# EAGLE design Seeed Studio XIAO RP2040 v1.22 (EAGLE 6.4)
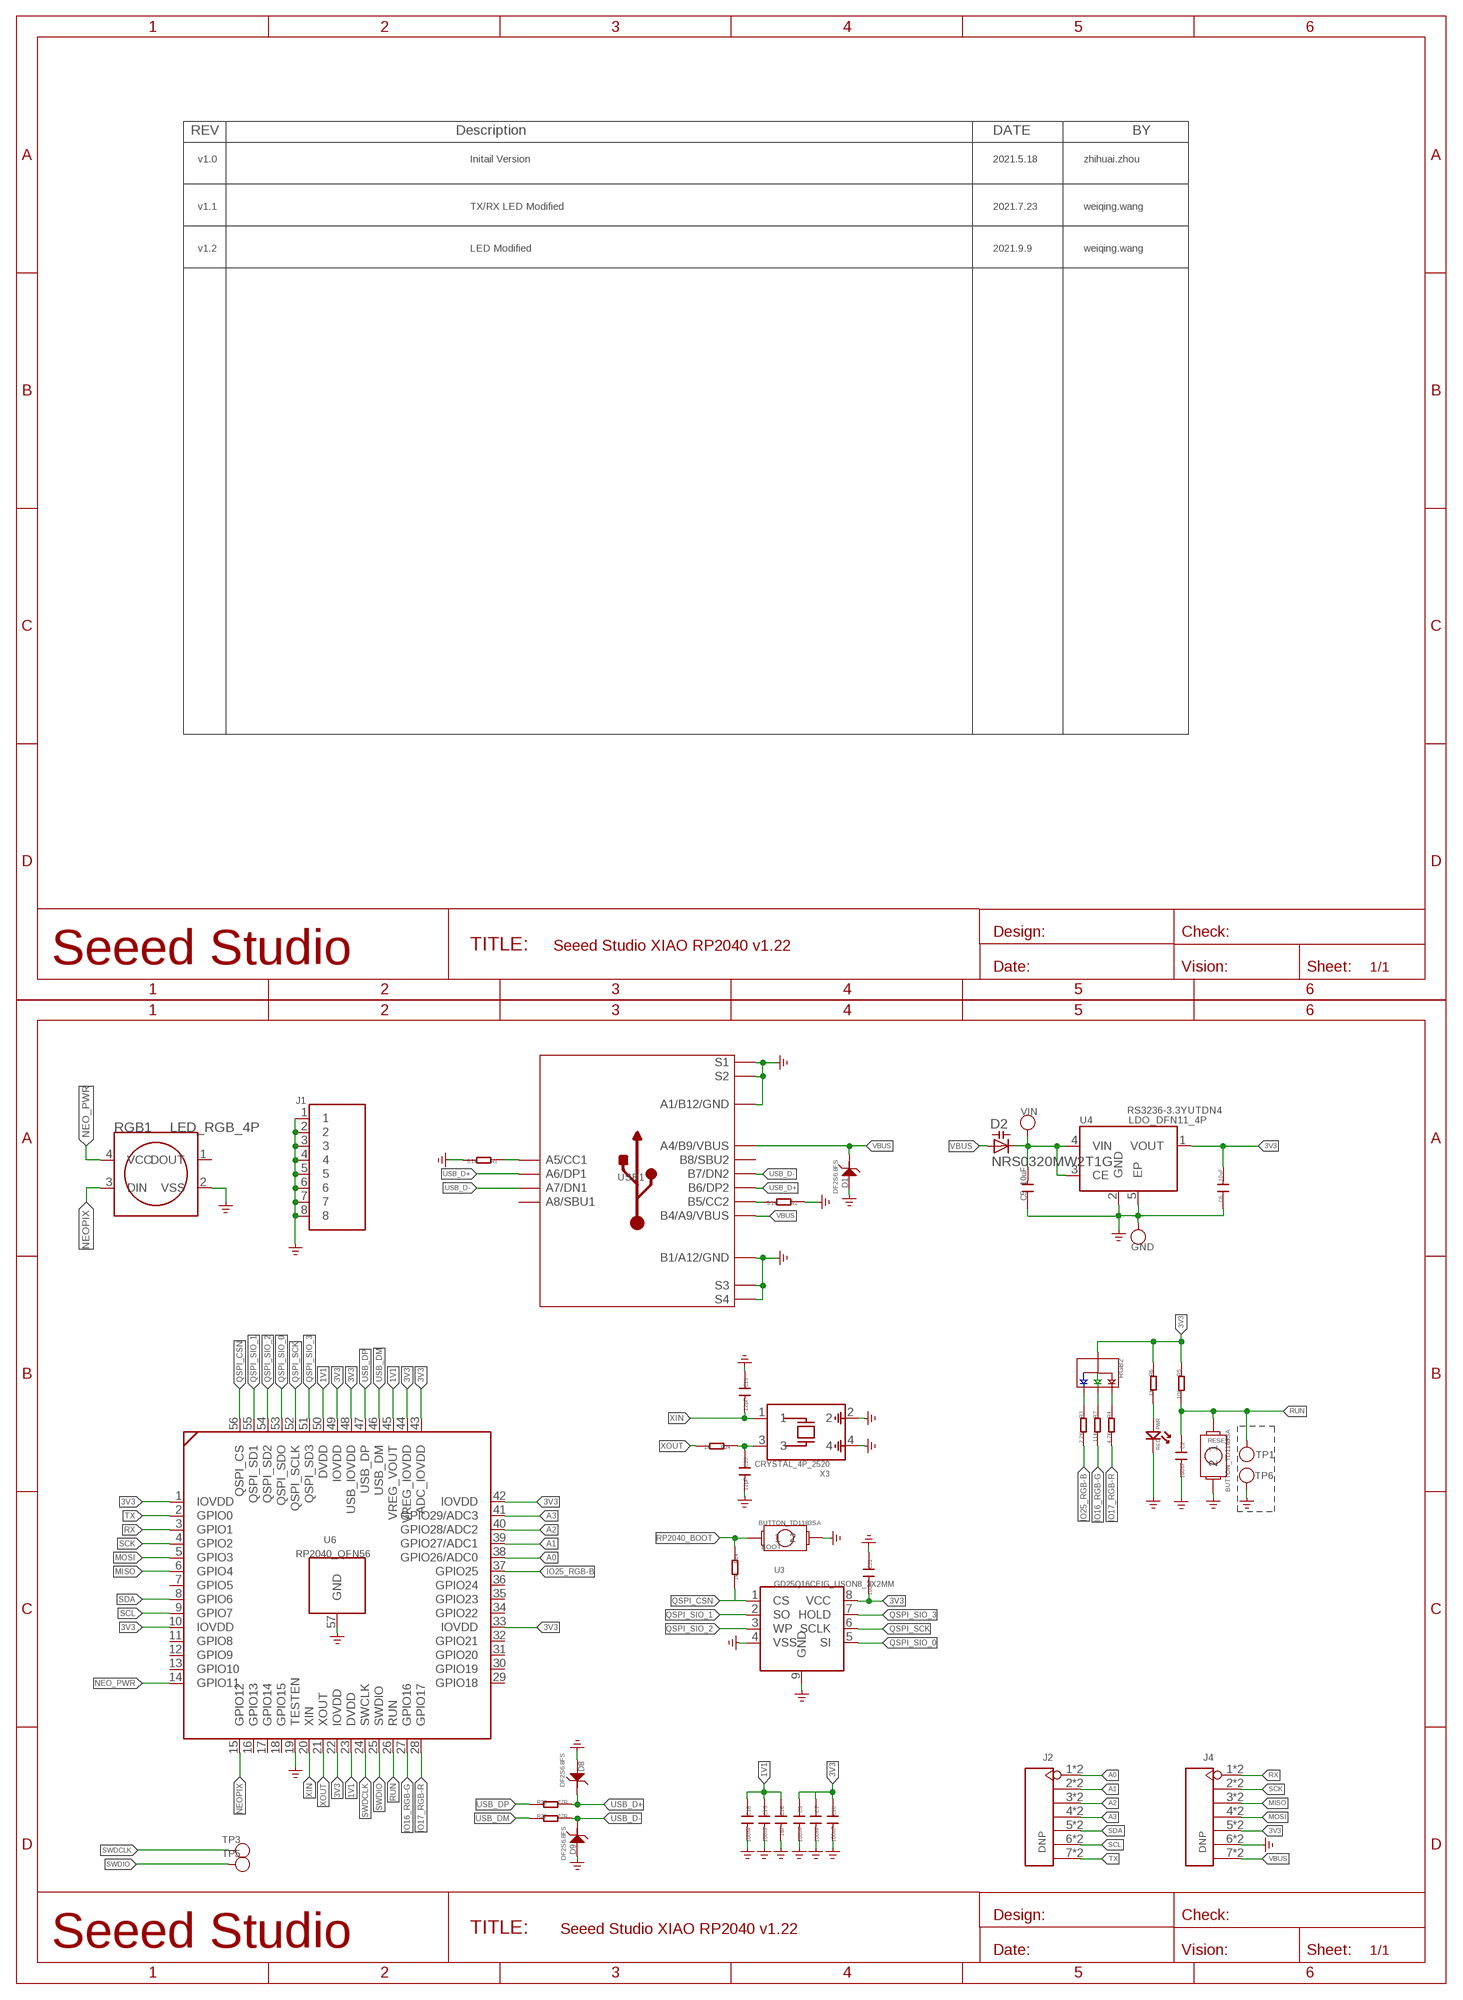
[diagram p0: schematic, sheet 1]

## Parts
BOOT  BUTTON_TD1183SA  [BUTTON_TD1183SA]
C2  100nF  CAP\0201NNS  [0201_NORMAL\NOSILK]
C3  100nF  CAP\0201NNS  [0201_NORMAL\NOSILK]
C5  10uF  C-0402  [C0402]
C6  10uF  C-0402  [C0402]
C7  100nF  CAP\0201NNS  [0201_NORMAL\NOSILK]
C10  100nF  CAP\0201NNS  [0201_NORMAL\NOSILK]
C15  100nF  CAP\0201NNS  [0201_NORMAL\NOSILK]
C16  1uF  CAP\0201NNS  [0201_NORMAL\NOSILK]
C18  100nF  CAP\0201NNS  [0201_NORMAL\NOSILK]
C19  12pF  CAP\0201NNS  [0201_NORMAL\NOSILK]
C20  12pF  CAP\0201NNS  [0201_NORMAL\NOSILK]
C21  100nF  CAP\0201NNS  [0201_NORMAL\NOSILK]
D1  DF2S6.8FS  D-ESD-2P'DF2S6.8FS'  [SOD-923]
D2  NRS0320MW2T1G  DIODE_CAPACITANCE-SOD523  [SOD523]
D8  DF2S6.8FS  D-ESD-2P'DF2S6.8FS'  [SOD-923]
D9  DF2S6.8FS  D-ESD-2P'DF2S6.8FS'  [SOD-923]
GND  TEST-POINT'4080'  [TP-80X40MIL]
J1  SHIELDING-COVER-XIAO_RP2040_PRD  [SHIELDING-COVER_XIAO_RP2040_PRD]
J2  DNP  HEADER-7P-HALF-HOLE-2.54  [H7-HALF-HOLE-2.54]
J4  DNP  HEADER-7P-HALF-HOLE-2.54  [H7-HALF-HOLE-2.54]
PWR  RED  LED-0402  [LED-0402]
R1  5.1k  R-0201  [R0201]
R2  5.1k  R-0201  [R0201]
R3  2.2K  R-0201  [R0201]
R4  4.7K  R-0201  [R0201]
R5  10k  R-0201  [R0201]
R6  1k  R-0201  [R0201]
R7  11K  R-0201  [R0201]
R14  1k  R-0201  [R0201]
R22  27R  R-0201  [R0201]
R23  27R  R-0201  [R0201]
R24  1k  R-0201  [R0201]
RESET  BUTTON_TD1183SA  [BUTTON_TD1183SA]
RGB1  LED_RGB_4P  [LED_RGB_2427]
RGB2  LED_RGB_4P-1010  [1010-4P]
TP1  TEST-POINT'4545'  [TP-D45MIL]
TP3  TEST-POINT'4545'  [TP-D45MIL]
TP5  TEST-POINT'4545'  [TP-D45MIL]
TP6  TEST-POINT'4545'  [TP-D45MIL]
U3  GD25Q16CEIG_USON8_3X2MM  [GD25Q16CEIG_USON8_3X2MM]
U4  LDO_DFN11_4P  [LDO_DFN1*1_4P]
U6  RP2040_QFN56  [RP2040_QFN56]
USB1  USB2.0-TYPE-C  [USB2.0-TYPE-C]
VIN  TEST-POINT'4080'  [TP-80X40MIL]
X3  CRYSTAL_4P_2520  [CRYSTAL_4P_2520]

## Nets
1V1: C15.1 C16.1 C18.1 U6.23(DVDD) U6.45(VREG_VOUT) U6.50(DVDD)
3V3: C3.1 C6.2 C7.1 C10.1 C21.2 J4.5 J4.17 R5.1 R6.1 RGB2.+ U3.8(VCC) U4.1(VOUT) U6.1(IOVDD) U6.10(IOVDD) U6.22(IOVDD) U6.33(IOVDD) U6.42(IOVDD) U6.43(ADC_IOVDD) U6.44(VREG_IOVDD) U6.48(USB_IOVDD) U6.49(IOVDD)
A0: J2.1 J2.13 U6.38(GPIO26/ADC0)
A1: J2.2 J2.14 U6.39(GPIO27/ADC1)
A2: J2.3 J2.15 U6.40(GPIO28/ADC2)
A3: J2.4 J2.16 U6.41(GPIO29/ADC3)
GND: BOOT.2 C2.2 C3.2 C5.1 C6.1 C7.2 C10.2 C15.2 C16.2 C18.2 C19.1 C20.2 C21.1 D1.2 D8.2 D9.2 GND.1(T) J1.1 J1.2 J1.3 J1.4 J1.5 J1.6 J1.7 J1.8 J4.6 J4.18 PWR.- R1.2 R2.1 RESET.2 RGB1.2(VSS) TP6.T U3.4(VSS) U3.9(GND) U4.2(GND) U4.5(EP) U6.19(TESTEN) U6.57(GND) USB1.A1_B12(A1/B12/GND) USB1.B1_A12(B1/A12/GND) USB1.S1 USB1.S2 USB1.S3 USB1.S4 USB1.S5(S1) USB1.S6(S2) X3.2 X3.4 ; supply symbol labelled GND_POWER
IO16_RGB-G: R7.2 U6.27(GPIO16)
IO17_RGB-R: R4.2 U6.28(GPIO17)
IO25_RGB-B: R3.2 U6.37(GPIO25)
MISO: J4.3 J4.15 U6.6(GPIO4)
MOSI: J4.4 J4.16 U6.5(GPIO3)
N$1: R1.1 USB1.A5(A5/CC1)
N$2: R2.2 USB1.B5(B5/CC2)
N$3: R3.1 RGB2.B-
N$4: R7.1 RGB2.G-
N$6: R4.1 RGB2.R-
N$8: C20.1 R24.1 X3.3
N$16: PWR.+ R6.2
NEO_PWR: RGB1.4(VCC) U6.14(GPIO11)
NEOPIX: RGB1.3(DIN) U6.15(GPIO12)
QSPI_CSN: R14.2 U3.1(CS) U6.56(QSPI_CS)
QSPI_SCK: U3.6(SCLK) U6.52(QSPI_SCLK)
QSPI_SIO_0: U3.5(SI) U6.53(QSPI_SDO)
QSPI_SIO_1: U3.2(SO) U6.55(QSPI_SD1)
QSPI_SIO_2: U3.3(WP) U6.54(QSPI_SD2)
QSPI_SIO_3: U3.7(HOLD) U6.51(QSPI_SD3)
RP2040_BOOT: BOOT.1 R14.1
RUN: C2.1 R5.2 RESET.1 TP1.T U6.26(RUN)
RX: J4.1 J4.13 U6.3(GPIO1)
SCK: J4.2 J4.14 U6.4(GPIO2)
SCL: J2.6 J2.18 U6.9(GPIO7)
SDA: J2.5 J2.17 U6.8(GPIO6)
SWDCLK: TP3.T U6.24(SWCLK)
SWDIO: TP5.T U6.25(SWDIO)
TX: J2.7 J2.19 U6.2(GPIO0)
USB_D+: D8.1 R23.2 USB1.A6(A6/DP1) USB1.B6(B6/DP2)
USB_D-: D9.1 R22.2 USB1.A7(A7/DN1) USB1.B7(B7/DN2)
USB_DM: R22.1 U6.46(USB_DM)
USB_DP: R23.1 U6.47(USB_DP)
VBUS: D1.1 D2.A J4.7 J4.19 USB1.A4_B9(A4/B9/VBUS) USB1.B4_A9(B4/A9/VBUS)
VIN: C5.2 D2.C U4.3(CE) U4.4(VIN) VIN.1(T)
XIN: C19.2 U6.20(XIN) X3.1
XOUT: R24.2 U6.21(XOUT)
Unconnected: RGB1.1(DOUT) U6.7(GPIO5) U6.11(GPIO8) U6.12(GPIO9) U6.13(GPIO10) U6.16(GPIO13) U6.17(GPIO14) U6.18(GPIO15) U6.29(GPIO18) U6.30(GPIO19) U6.31(GPIO20) U6.32(GPIO21) U6.34(GPIO22) U6.35(GPIO23) U6.36(GPIO24) USB1.A8(A8/SBU1) USB1.B8(B8/SBU2)

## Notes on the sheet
- v1.0 | Initail Version | 2021.5.18 | zhihuai.zhou
- v1.1 | TX/RX LED Modified | 2021.7.23 | weiqing.wang
- v1.2 | LED Modified | 2021.9.9 | weiqing.wang
- RS3236-3.3YUTDN4

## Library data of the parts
BOOT RESET = BUTTON_TD1183SA:BUTTON_TD1183SA: 德艺隆:TD-1183SA/311020740
C2 C3 C7 C10 C15 C16 C18-C21 = Seeed-Discrete:CAP: Ceramic Capacitors
C5 C6 = XIAO RP2040 PRD v1.0:C*: Ceramic Capacitors
D1 D8 D9 = Discrete-new:D-ESD-2P: SOD-923:304060009;SOD-123:304060001
D2 = XIAO RP2040 PRD v1.0:DIODE_CAPACITANCE-: Capacity DIODE
GND VIN = Discrete-new:TEST-POINT
J1 = XIAO RP2040 PRD v1.0:SHIELDING-COVER-XIAO_RP2040_PRD
J2 J4 = Connector-new:HEADER-7P-HALF-HOLE
PWR = Discrete-small:LED
R1-R7 R14 R22-R24 = XIAO RP2040 PRD v1.0:R*
RGB1 = XIAO RP2040 PRD v1.0:LED_RGB_4P
RGB2 = Seeed-Discrete:LED_RGB_4P
TP1 TP3 TP5 TP6 = Discrete-new:TEST-POINT; PARTNO: DNP
U3 = FLASH_GD25Q16CEIG_2:GD25Q16CEIG_USON8_3X2MM
U4 = LDO_DFN1X1_4P:LDO_DFN1*1_4P
U6 = RP2040_QFN56:RP2040_QFN56
USB1 = USB C:USB2.0-TYPE-C
X3 = CRYSTAL_4P:CRYSTAL_4P_2520

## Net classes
1 power: width 0.152 mm, drill 0.152 mm, clearance 0.152 mm
2 gnd: width 0.152 mm, drill 0.152 mm, clearance 0.152 mm
3 usbvcc: width 0.152 mm, drill 0.152 mm, clearance 0.152 mm

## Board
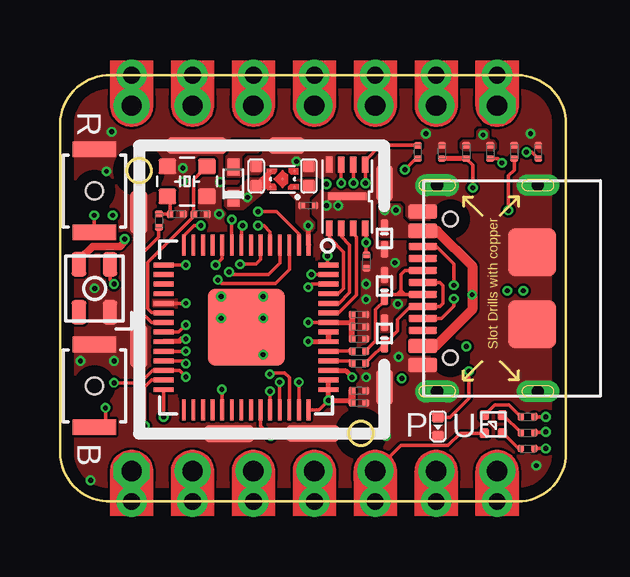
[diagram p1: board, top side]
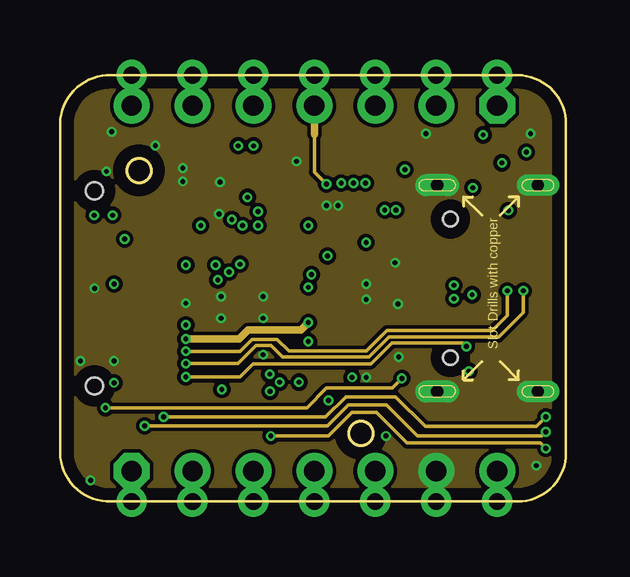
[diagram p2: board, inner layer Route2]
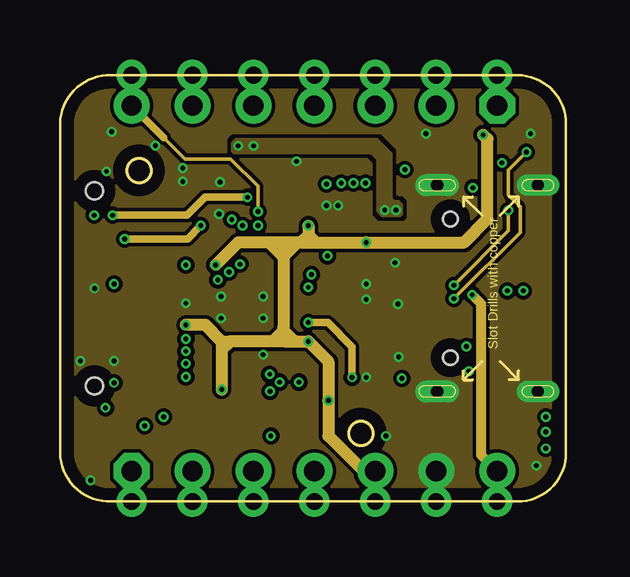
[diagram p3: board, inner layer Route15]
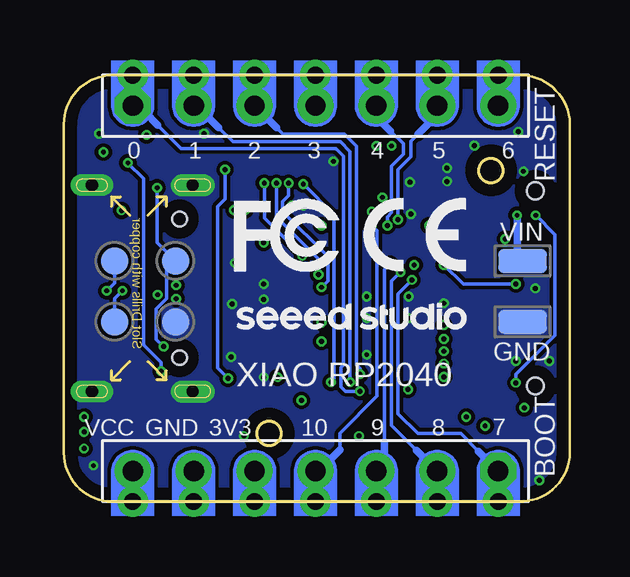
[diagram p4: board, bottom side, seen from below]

Size 21.1 x 17.78 mm. Coordinates in mm from the lower left corner, seen from the top.
Outline: 2.13,0 19.07,0 arc90 21.1,2.03 21.1,15.75 arc90 19.07,17.78 2.13,17.78 arc90 0,15.75 0,2.03 arc90 2.13,0
Copper layers (1+2*15+16): Top 0.035mm / dielectric 0.2mm / Route2 0.0175mm / dielectric 1.1mm / Route15 0.0175mm / dielectric 0.2mm / Bottom 0.035mm
Design rules "SeeedStudio_2layer_DRU_no_angle_20140221 *": minimum track width 1mil, minimum drill 8mil, track to track 4mil, track to pad 4mil, pad to pad 6mil, via to via 4mil, smd to smd 0mil, copper to edge 20mil, drill to drill 10mil, minimum pad ring 4mil, minimum via ring 4mil, stop-mask expansion 2mil, vias tented up to drill 25mil, thermal gap 0mil
tRestrict: area 4.9,4.3 to 10.6,10.2

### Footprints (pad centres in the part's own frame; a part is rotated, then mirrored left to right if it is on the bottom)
BUTTON_TD1183SA = smd 0.65 x 1.8: 1 -1.725,0; 2 1.725,0 | hole 0.7: 0,0
0201_NORMAL\NOSILK = smd 0.279 x 0.318: 1 -0.279,0; 2 0.279,0
C0402 = smd 0.508 x 0.508: 1 -0.406,0; 2 0.406,0
SOD-923 = smd 0.7 x 0.3: 1 -0.45,0; 2 0.45,0
SOD523 = smd 0.7 x 0.5: A 0.7,0; C -0.6,0
TP-80X40MIL = smd 2.032 x 1.016: 1 0,0
SHIELDING-COVER_XIAO_RP2040_PRD = smd 0.7 x 1.778: 1 -4.953,3.556; 2 -4.953,-2.032 | smd 2.032 x 0.7: 3 -1.18,-5.673 | smd 2.2 x 0.7: 4 2.29,-5.668 | smd 0.7 x 1.5: 5 5.283,-3.737; 6 5.283,4.772 | smd 1.5 x 0.7: 7 1.216,6.332 | smd 2.5 x 0.7: 8 -2.54,6.332 | hole 1: -4.953,5.3; 4.3,-5.672
H7-HALF-HOLE-2.54 = drill 0.85 pad 1.5 octagon: 1 0,7.62 | drill 0.85 pad 1.5: 2 0,5.08; 3 0,2.54; 4 0,0; 5 0,-2.54; 6 0,-5.08; 7 0,-7.62 | drill 0.7 pad 1.27: 13 -1.27,7.62; 14 -1.27,5.08; 15 -1.27,2.54; 16 -1.27,0; 17 -1.27,-2.54; 18 -1.27,-5.08; 19 -1.27,-7.62
LED-0402 = smd 0.385 x 0.508: + -0.383,0; - 0.383,0
R0201 = smd 0.279 x 0.318: 1 -0.279,0; 2 0.279,0
LED_RGB_2427 = smd 1 x 0.6: 1 1,-0.65; 2 1,0.65; 3 -1,0.65; 4 -1,-0.65
1010-4P = smd 0.4 x 0.4: + 0.375,0.375; B- -0.375,0.375; G- -0.375,-0.375; R- 0.375,-0.375
TP-D45MIL = smd 1.143 x 1.143: T 0,0
GD25Q16CEIG_USON8_3X2MM = smd 0.65 x 0.3: 1 -1.33,0.75; 2 -1.33,0.25; 3 -1.33,-0.25; 4 -1.33,-0.75; 5 1.33,-0.75; 6 1.33,-0.25; 7 1.33,0.25; 8 1.33,0.75 | smd 0.3 x 1.6: 9 0,0
LDO_DFN1*1_4P = smd 0.1 x 0.1: 1 -0.33,-0.5; 2 0.33,-0.5; 3 0.33,0.51; 4 -0.33,0.5; 5 0,0
RP2040_QFN56 = smd 0.875 x 0.2: 1 -3.438,2.6; 2 -3.438,2.2; 3 -3.438,1.8; 4 -3.438,1.4; 5 -3.438,1; 6 -3.438,0.6; 7 -3.438,0.2; 8 -3.438,-0.2; 9 -3.438,-0.6; 10 -3.438,-1; 11 -3.438,-1.4; 12 -3.438,-1.8; 13 -3.438,-2.2; 14 -3.438,-2.6; 29 3.438,-2.6; 30 3.438,-2.2; 31 3.438,-1.8; 32 3.438,-1.4; 33 3.438,-1; 34 3.438,-0.6; 35 3.438,-0.2; 36 3.438,0.2; 37 3.438,0.6; 38 3.438,1; 39 3.438,1.4; 40 3.438,1.8; 41 3.438,2.2; 42 3.438,2.6 | smd 0.2 x 0.875: 15 -2.6,-3.438; 16 -2.2,-3.438; 17 -1.8,-3.438; 18 -1.4,-3.438; 19 -1,-3.438; 20 -0.6,-3.438; 21 -0.2,-3.438; 22 0.2,-3.438; 23 0.6,-3.438; 24 1,-3.438; 25 1.4,-3.438; 26 1.8,-3.438; 27 2.2,-3.438; 28 2.6,-3.438; 43 2.6,3.438; 44 2.2,3.438; 45 1.8,3.438; 46 1.4,3.438; 47 1,3.438; 48 0.6,3.438; 49 0.2,3.438; 50 -0.2,3.438; 51 -0.6,3.438; 52 -1,3.438; 53 -1.4,3.438; 54 -1.8,3.438; 55 -2.2,3.438; 56 -2.6,3.438 | smd 3.2 x 3.2: 57 0,0
USB2.0-TYPE-C = smd 1.2 x 0.6: A1_B12 0.05,3.2; A4_B9 0.05,2.4; B1_A12 0.05,-3.2; B4_A9 0.05,-2.4 | smd 1.2 x 0.3: A5 0.05,1.25; A6 0.05,0.25; A7 0.05,-0.25; A8 0.05,-1.25; B5 0.05,-1.75; B6 0.05,-0.75; B7 0.05,0.75; B8 0.05,1.75 | drill 0.508 pad 0.889 long: S1 -4.75,4.3; S2 -4.75,-4.3 | drill 0.508 pad 0.914 long: S3 -0.55,4.3; S4 -0.55,-4.3 | smd 2 x 2: S5 -4.5,1.5; S6 -4.5,-1.5 | hole 0.6: -1.1,-2.89; -1.1,2.89
CRYSTAL_4P_2520 = smd 0.75 x 0.65: 1 -0.825,-0.625; 2 0.825,-0.625; 3 0.825,0.625; 4 -0.825,0.625

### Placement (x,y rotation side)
BOOT  1.44,4.83 90 top
C2  15.93,14.58 90 top
C3  10.36,12.34 0 top
C5  8.18,13.58 270 top
C6  10.38,13.58 270 top
C7  12.46,4.62 0 top
C10  12.46,4.11 0 top
C15  12.46,7.8 0 top
C16  12.46,6.78 0 top
C18  12.46,7.29 0 top
C19  5.87,11.97 180 top
C20  4.87,11.97 0 top
C21  12.78,10.01 90 top
D1  13.53,10.97 270 top
D2  7.23,13.25 90 top
D8  13.53,8.99 90 top
D9  13.53,7.01 90 top
GND  1.97,7.49 0 bottom
J1  8.25,8.51 0 top
J2  10.61,16.51 270 top
J4  10.61,1.27 90 top
PWR  15.77,3.12 270 top
R1  19.94,14.58 90 top
R2  18.94,14.58 270 top
R3  19.5,2.21 0 top
R4  19.5,3.53 0 top
R5  16.93,14.58 270 top
R6  17.94,14.58 270 top
R7  19.5,2.87 0 top
R14  14.93,14.58 90 top
R22  12.46,5.77 0 top
R23  12.46,6.27 0 top
R24  4.12,11.71 270 top
RESET  1.44,12.95 90 top
RGB1  1.44,8.89 270 top
RGB2  18.08,3.22 180 top
TP1  16.45,10.03 0 bottom
TP3  18.99,7.49 0 bottom
TP5  18.99,10.03 0 bottom
TP6  16.45,7.49 0 bottom
U3  11.98,12.73 270 top
U4  9.29,13.44 90 top
U6  7.76,7.26 270 top
U$4  [LOGO-SEEED-NEW-1X9.6MM]  13.91,7.11 0 bottom
USB1  15.18,8.89 180 top
VIN  1.97,10.03 180 bottom
X3  5.3,13.35 180 top

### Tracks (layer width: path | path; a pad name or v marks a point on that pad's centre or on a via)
1V1  (via drill 0.2 pad 0.41)
  Top 0.152: v10.36,7.46 U6.50
  Top 0.203: U6.50 12.18,7.46 C18.1 | U6.23 4.34,6.68 4.97,6.68 5.07,6.78 v5.25,6.78 | U6.45 11.9,5.46 v12.18,5.18
  Top 0.254: C15.1 C18.1 C16.1
  Route2 0.305: v5.25,6.78 7.48,6.78 7.85,7.16 10.05,7.16 v10.36,7.46
  Route15 0.305: v12.18,5.18 12.18,6.45 11.17,7.46 v10.36,7.46
3V3  (via drill 0.2 pad 0.41)
  Top 0.152: U6.22 4.95,7.06 v5.25,7.37 | v11.19,4.22 10.8,3.83 U6.42 | U3.8 12.77,11.36 v12.77,10.8 12.77,10.3 C21.2 | v6.75,4.67 6.76,4.66 U6.33 | v6.49,9.87 6.76,10.14 U6.10 | RGB2.+ 16.69,2.85 16.18,2.34 14.22,2.34 J4.5
  Top 0.203: U6.48 U6.49 11.2,6.68 v10.36,6.68 | U6.44 U6.43 v11.19,4.22 12.08,4.22 C10.1 | U6.42 10.38,3.84 | U6.1 v10.36,11.51
  Top 0.254: J4.5 J4.17
  Top 0.305: C10.1 C7.1
  Route15 0.305: 8.59,10.8 9.26,10.14 9.31,10.14 9.37,10.14 10.04,10.8 | 8.59,6.68 8.73,6.68 9.31,7.26 9.85,6.73 9.85,6.68
  Route15 0.508: 9.34,6.68 9.85,6.68 v10.36,6.68 11.19,5.84 v11.19,4.22 11.19,2.73 12.66,1.27 J4.5 | 9.34,6.68 8.59,6.68 7.1,6.68 | 6.75,6.68 7.1,6.68 | 10.36,10.8 10.67,10.8 | v10.36,11.51 10.36,11.12 | 10.36,11.12 10.36,10.8 | 10.04,10.8 10.36,10.8 | 10.04,10.8 9.31,10.8 | 9.31,10.8 8.59,10.8 7.43,10.8 v6.49,9.87 | 7.1,6.68 6.75,6.33 | 10.04,10.8 10.36,11.12 | 10.36,11.12 10.67,10.8 | 9.31,10.8 9.31,10.14 9.31,7.26 9.31,6.71 9.34,6.68 | 6.75,6.68 6.75,6.33 | v17.65,15.29 17.82,15.11 17.82,11.77 16.85,10.8 v12.77,10.8 10.67,10.8 | v5.25,7.37 6.06,7.37 6.75,6.68 | 6.75,6.33 v6.75,4.67
  pour Top: 9.5,13.06 9.9,13.45 10.63,13.45 10.72,13.36 10.72,12.99 10.38,12.65 10.38,11.89 10.62,11.65 10.62,11.38 10.51,11.26 10.22,11.26 9.85,11.63 9.85,12.55 9.5,12.89
  pour Top: 17.3,15.07 16.79,15.07 16.67,14.95 16.67,14.76 16.79,14.63 18.09,14.63 18.22,14.76 18.22,14.94 18.09,15.06 17.99,15.06 17.91,15.14 17.91,15.43 17.81,15.53 17.47,15.53 17.37,15.43 17.37,15.14
A0  (via drill 0.2 pad 0.41)
  Top 0.152: v8.76,4.6 U6.38
  Top 0.254: J2.1 J2.13
  Bottom 0.152: 17.19,15.7 16.21,14.72 9.75,14.72 9.44,14.41 9.44,5.7 9.54,5.6 9.54,4.79 9.35,4.6 9,4.6 v8.76,4.6
  Bottom 0.305: 17.19,15.7 17.72,16.23 17.95,16.23 J2.1
A1  (via drill 0.2 pad 0.41)
  Top 0.152: v9.16,4.98 U6.39
  Top 0.254: J2.2 J2.14
  Bottom 0.102: J2.2 15.69,16
  Bottom 0.152: 14.65,15.6 14.05,15 9.57,15 9.16,14.59 v9.16,4.98
  Bottom 0.305: 14.65,15.6 15.08,16.03 15.66,16.03 15.69,16
A2  (via drill 0.2 pad 0.41)
  Top 0.152: U6.40 9.57,5.17 9.36,5.37 8.81,5.37 v8.75,5.31
  Top 0.254: J2.3 J2.15
  Bottom 0.152: 12.34,15.7 12.34,15.65 | v8.75,5.31 8.75,5.55 8.9,5.7 8.9,14.82 9.39,15.32 11.96,15.32 12.24,15.6
  Bottom 0.305: J2.3 12.34,15.7 12.24,15.6
A3  (via drill 0.2 pad 0.41)
  Top 0.152: v9.96,4.98 U6.41
  Top 0.254: J2.4 J2.16
  Route2 0.152: 10.61,15.32 10.61,13.74 v11.12,13.23
  Route2 0.305: J2.4 10.61,15.32
  Bottom 0.152: v9.96,4.98 9.83,5.11 9.83,11.95 v11.12,13.23
GND  (via drill 0.2 pad 0.41)
  Top 0.152: v5.25,8.27 v5.25,8.26 U6.19
  Top 0.305: U6.57 7.76,6.83 v8.48,6.12
  other vias: 8.48,7.65 6.72,7.65 8.48,8.55 1.44,8.89 0.86,5.87 2.25,5.87 1.94,13.77 2.15,15.42 3.98,14.85 6.68,13.32 11.12,12.34 11.6,12.34 12.77,8.43 12.77,9.07 12.77,5.18 1.28,0.89 19.87,1.5 13.59,2.73 19.63,15.34 15.26,15.34 6.72,8.55 5.12,13.91 9.86,14.19 14.13,6.03 14.09,8.24 13.98,9.96 6.63,11.99 5.12,13.35
  pour Top (rank 3, no thermals): -0.19,17.93 21.51,17.93 21.53,17.91 21.53,-0.28 3.88,-0.28 3.88,-0.91 2.08,-0.91 2.08,-0.25 -0.21,-0.25
  pour Route2 (isolate 0.152, rank 6, no thermals): -0.19,17.93 21.51,17.93 21.53,17.91 21.53,-0.28 3.88,-0.28 3.85,-1.24 2.08,-1.24 2.08,-0.25 -0.21,-0.25
  pour Route15 (isolate 0.152, rank 6, no thermals): -0.19,17.93 21.51,17.93 21.53,17.91 21.53,-0.28 3.88,-0.28 3.85,-1.57 2.08,-1.57 2.08,-0.25 -0.21,-0.25
  pour Bottom (isolate 0.152, rank 6, no thermals): -0.19,17.93 21.51,17.93 21.53,17.91 21.53,-0.28 3.88,-0.28 3.85,-1.93 2.08,-1.93 2.08,-0.25 -0.21,-0.25
IO16_RGB-G  (via drill 0.2 pad 0.41)
  Top 0.152: U6.27 3.82,5.06 3.54,4.78 v3.54,3.15 | R7.2 20.23,2.87 v20.26,2.91
  Route2 0.152: v3.54,3.15 11.16,3.15 12.03,4.02 13.62,4.02 14.9,2.74 20.1,2.74 v20.26,2.91
IO17_RGB-R  (via drill 0.2 pad 0.41)
  Top 0.152: U6.28 v4.33,3.54 v4.32,3.53 | R4.2 v20.26,3.54 v20.26,3.53
  Route2 0.152: v4.32,3.53 11.08,3.53 11.92,4.37 13.99,4.37 15.23,3.12 19.86,3.12 v20.26,3.53
IO25_RGB-B  (via drill 0.2 pad 0.41)
  Top 0.152: U6.37 8.36,3.16 v8.79,2.73 | R3.2 v20.26,2.21
  Route2 0.152: v8.79,2.73 11.19,2.73 12.17,3.71 13.2,3.71 14.47,2.44 20.03,2.44 v20.26,2.21
MISO  (via drill 0.2 pad 0.41)
  Top 0.152: U6.6 8.37,10.69 8.37,10.08 8.19,9.9 v7.51,9.9
  Top 0.254: J4.3 J4.15
  Bottom 0.152: v7.51,9.9 7.74,9.67 7.74,2.49
  Bottom 0.305: J4.3 7.74,1.6 7.74,2.49
MOSI  (via drill 0.2 pad 0.41)
  Top 0.152: U6.5 8.76,11.24 8.5,11.51 v8.26,11.51
  Top 0.254: J4.4 J4.16
  Bottom 0.152: 9.59,2.15 9.59,2.85 8.04,4.39 8.04,11.29 v8.26,11.51
  Bottom 0.305: 9.59,2.15 10.47,1.27 J4.4
N$1  (via drill 0.2 pad 0.41)
  Top 0.152: USB1.A5 15.91,7.64 16.43,8.15 v16.43,8.46 | R1.1 19.68,14.57 v19.45,14.57
  Route15 0.152: v16.43,8.46 19.19,11.23 19.19,12.29 18.7,12.79 18.7,13.82 v19.45,14.57
N$2  (via drill 0.2 pad 0.41)
  Top 0.152: USB1.B5 15.69,10.64 16.43,9.91 v16.43,9.02 | v18.7,12.14 18.7,13.59 18.94,13.83 R2.2
  Route15 0.152: v16.43,9.02 18.7,11.29 v18.7,12.14
N$3
  Top 0.152: RGB2.B- 18.48,2.85 19.12,2.21 R3.1
N$4
  Top 0.152: RGB2.G- 18.5,3.6 R7.1
N$6
  Top 0.152: 17.7,3.64 RGB2.R- 18.14,4.04 18.72,4.04 R4.1
N$8
  Top 0.152: R24.1 4.57,11.99 C20.1 4.59,12.61 X3.3
N$16  (via drill 0.2 pad 0.41)
  Top 0.152: v18.43,14.12 18.25,14.3 R6.2 | v17.05,5.44 17.05,4.31 16.25,3.51 PWR.+
  Bottom 0.152: v18.43,14.12 17.77,13.46 17.77,6.53 17.05,5.8 v17.05,5.44
NEO_PWR  (via drill 0.2 pad 0.41)
  Top 0.152: RGB1.4 0.79,10.07 | U6.14 5.16,11.08 5.59,11.51 v5.87,11.51
  Top 0.305: 0.79,10.07 1.37,10.64 2.5,10.64 2.7,10.84 v2.7,10.95
  Route15 0.305: v2.7,10.95 5.31,10.95 v5.87,11.51
NEOPIX  (via drill 0.2 pad 0.41)
  Top 0.152: v5.25,9.87 U6.15 | 2.09,9.49 RGB1.3 2.09,9.23 v2.25,9.07
  Bottom 0.152: v2.25,9.07 4.45,9.07 v5.25,9.87
QSPI_CSN  (via drill 0.2 pad 0.41)
  Top 0.152: v11.16,10.25 11.15,10.24 11.15,9.92 U6.56 | R14.2 13.37,14.86 12.73,14.22 U3.1 12.74,14.04 v12.74,13.28
  Bottom 0.152: v11.16,10.25 12.74,11.83 v12.74,13.28
QSPI_SCK
  Top 0.152: U3.6 11.73,11.05 12.08,10.7 12.08,8.72 11.63,8.26 U6.52
QSPI_SIO_0
  Top 0.152: 11.28,11.23 11.28,11.35 U3.5 11.23,11.01 11.83,10.41 11.83,8.89 11.6,8.66 U6.53
QSPI_SIO_1  (via drill 0.2 pad 0.41)
  Top 0.152: v10.48,9.47 v10.49,9.46 U6.55 | v12.24,13.28 U3.2
  Bottom 0.152: 12.24,13.31 v12.24,13.28 12.24,11.86 10.48,10.11 v10.48,9.47
QSPI_SIO_2  (via drill 0.2 pad 0.41)
  Top 0.152: v11.73,13.28 U3.3 | v10.36,8.94 10.48,9.06 U6.54
  Bottom 0.152: v11.73,13.28 11.73,12.76 11.98,12.5 11.98,12.09 10.1,10.21 10.1,9.2 v10.36,8.94
QSPI_SIO_3
  Top 0.152: U6.51 11.61,7.86 12.37,8.62 12.37,11.04 12.23,11.18 U3.7
RP2040_BOOT  (via drill 0.2 pad 0.41)
  Top 0.152: R14.1 14.84,14.3 v14.38,13.84 | v1.9,3.91 1.9,2.97 1.95,2.92 1.62,2.92 BOOT.1
  Route2 0.152: v1.9,3.91 10.29,3.91 11.12,4.74 13.86,4.74 v14.25,5.13
  Bottom 0.152: v14.25,5.13 14.7,5.58 14.7,12.29 14.38,12.61 v14.38,13.84
RUN  (via drill 0.2 pad 0.41)
  Top 0.152: RESET.1 1.43,11.24 v1.43,11.94 | R5.2 17.21,14.02 v17.21,13.08 | v2.25,4.95 3.35,4.95 3.86,5.46 U6.26 4.98,5.46 v5.25,5.19
  Top 0.203: R5.2 C2.1
  Route2 0.152: v16.95,6.46 16.81,6.6 13.84,6.6 12.97,5.74 8.06,5.74 7.51,5.19 v5.25,5.19
  Bottom 0.152: v17.21,13.08 17.21,10.79 TP1.T 16.81,9.68 16.81,8.46 17.25,8.02 17.25,6.77 v16.95,6.46 | v1.43,11.94 0.63,11.14 0.63,6.93 2.25,5.31 v2.25,4.95
RX  (via drill 0.2 pad 0.41)
  Top 0.152: v6.58,9.25 6.74,9.09 8.98,9.09 9.57,9.68 U6.3 | J4.1 2.99,0.33
  Top 0.254: J4.1 J4.13
  Bottom 0.152: 3.81,2.09 4.55,2.83 6.34,2.83 7.17,3.66 7.17,8.66 v6.58,9.25 | v6.58,9.25
  Bottom 0.305: J4.1 3.81,2.09
SCK  (via drill 0.2 pad 0.41)
  Top 0.152: v7.06,9.57 7.16,9.47 8.7,9.47 9.17,9.94 9.17,10.69 U6.4
  Top 0.254: J4.2 J4.14
  Bottom 0.152: 6.4,2.14 7.43,3.18 7.43,9.2 v7.06,9.57
  Bottom 0.305: J4.2 6.4,2.14
SCL  (via drill 0.2 pad 0.41)
  Top 0.152: U6.9 v7.16,11.76 v7.17,11.76
  Top 0.254: J2.6 J2.18
  Bottom 0.152: v7.17,11.76 7.17,13.84 6.63,14.38 6.63,15.02 6.33,15.33
  Bottom 0.305: J2.6 5.53,16.13 6.33,15.33
SDA  (via drill 0.2 pad 0.41)
  Top 0.152: U6.8 7.56,11.46 v7.61,11.51
  Top 0.254: J2.5 J2.17
  Bottom 0.152: v7.61,11.51 7.61,11.87 7.43,12.05 7.43,14 6.95,14.48 6.95,14.92 7.49,15.46
  Bottom 0.305: J2.5 8.07,16.04 7.49,15.46
SWDCLK  (via drill 0.2 pad 0.41)
  Top 0.152: v5.25,6.27 U6.24
  Route2 0.152: v5.25,6.27 7.52,6.27 8.01,6.76 9.05,6.76 9.54,6.27 10.14,6.27 12.78,6.27 13.63,7.13 18.03,7.13 18.66,7.76 v18.66,8.79
  Bottom 0.152: v18.66,8.79 18.99,8.46 TP3.T
SWDIO  (via drill 0.2 pad 0.41)
  Top 0.152: v5.25,5.75 5.14,5.86 U6.25
  Route2 0.152: v5.25,5.75 7.43,5.75 8.17,6.5 8.79,6.5 9.28,6.02 12.88,6.02 13.72,6.86 18.29,6.86 19.32,7.89 v19.32,8.79
  Bottom 0.152: v19.32,8.79 18.99,9.12 TP5.T
TX  (via drill 0.2 pad 0.41)
  Top 0.152: U6.2 9.96,11.15 9.02,12.09 v8.26,12.09 | 2.99,17.34 J2.19
  Top 0.381: J2.7 2.99,17.34
  Route15 0.152: v8.26,12.09 8.26,13.14 7.12,14.29 5.21,14.29 4.32,15.18
  Route15 0.305: J2.7 4.32,15.18
USB_D+
  Top 0.102: USB1.A6
  Top 0.152: USB1.B6 14.38,9.64 14.22,9.47 14.22,8.8 | R23.2 12.91,6.45 12.92,6.45 13.16,6.69 13.16,8 13.53,8.37 D8.1 13.62,8.54 13.72,8.64 | 13.63,8.64 13.72,8.64 | 13.72,8.64 13.92,8.64 14.05,8.64 | 14.05,8.64 14.22,8.64 | 14.22,8.64 14.38,8.64 | 14.38,8.64 USB1.A6 | 14.22,8.8 14.22,8.64 | 14.05,8.64 14.22,8.8 | 14.22,8.8 14.38,8.64
USB_D-
  Top 0.152: USB1.A7 15.84,9.14 15.97,9.02 15.97,8.26 15.85,8.14 USB1.B7 15.12,8.13 14.62,8.13 14.08,7.59 14.08,7.11 D9.1 12.92,5.94 12.91,5.94 R22.2
USB_DM
  Top 0.152: U6.46 12.09,5.86 R22.1
USB_DP
  Top 0.152: R23.1 11.2,6.27 U6.47
VBUS  (via drill 0.2 pad 0.41)
  Top 0.254: J4.7 J4.19
  Top 0.406: USB1.B4_A9 15.73,11.29 17.19,9.83 v17.19,8.62 17.19,8 15.69,6.5 15.14,6.5 USB1.A4_B9
  Route15 0.406: v17.19,8.62 17.56,8.26 17.56,1.94 J4.7
  other vias: 13.54,12.15 14.01,12.15 7.43,14.83 8.07,14.83
  pour Bottom (isolate 0.254, no thermals): 18.38,1.37 18,0.99 17.72,0.99
  pour Top: 13.38,11.01 15.64,11.01 15.69,11.06 15.69,11.53 15.65,11.57 14.53,11.57 14.31,11.8 14.31,12.08 14.31,12.28 14.18,12.41 13.42,12.41 13.28,12.27 13.28,11.98 13.28,11.11
  pour Top: 6.96,13.54 7.54,13.54 7.59,13.59 7.59,14.4 7.74,14.55 8.26,14.55 8.35,14.64 8.35,14.97 8.25,15.07 7.23,15.07 6.9,14.74 6.9,13.6
  pour Route15: 7.27,15.09 7.13,14.95 7.13,14.62 7.24,14.5 7.5,14.5 12.97,14.5 13.19,14.29 13.19,12.1 13.4,11.89 14.2,11.89 14.31,11.99 14.31,12.38 14.14,12.55 13.96,12.55 13.87,12.64 13.87,14.5 13.4,14.97 13.24,15.14 7.4,15.14 7.32,15.14
VIN  (via drill 0.2 pad 0.41)
  Top 0.152: C5.2 8.21,13.2 | C5.2 8.43,13.41 8.49,13.41 | 8.62,13.29 8.49,13.41 | 8.62,13.6 8.62,13.29 | U4.4 8.24,13.11 C5.2 | C5.2 8.35,13.17 | 8.35,13.17 8.5,13.17 8.62,13.29 | 8.49,13.41 8.49,13.31 8.35,13.17 | U4.3 8.7,13.69 8.7,13.2
  Top 0.254: U4.4 8.7,13.2 8.49,13.41 | U4.3 C5.2
  Route15 0.305: v2.2,11.94 5.3,11.94 6.05,12.69 v7.82,12.69
  Bottom 0.305: 2.3,9.98 2.28,10.01 1.52,10.01 | VIN.1 2.2,10.26 v2.2,11.94
  Bottom 0.406: VIN.1 1.31,10.03 1.34,10.01 1.52,10.01
  pour Top: 7.87,13.49 7.47,13.09 6.96,13.09 6.84,12.97 6.84,12.34 7.02,12.17 7.66,12.17 8.75,13.1 8.36,13.49
XIN
  Top 0.152: U6.20 4.32,7.87 3.83,7.87 3.65,8.05 3.65,9.97 5.59,11.9 C19.2 5.58,11.99 5.58,13.42 X3.1
XOUT
  Top 0.152: U6.21 3.83,7.46 3.35,7.95 3.35,10.26 4.12,11.04 R24.2

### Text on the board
tPlace: R | P | U | B
bNames: 6 | 5 | 4 | 3 | 2 | 1 | 0 | VIN | GND | XIAO RP2040 | 7 | 8 | 9 | 10 | 3V3 | GND | VCC
tTest: RESET | BOOT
